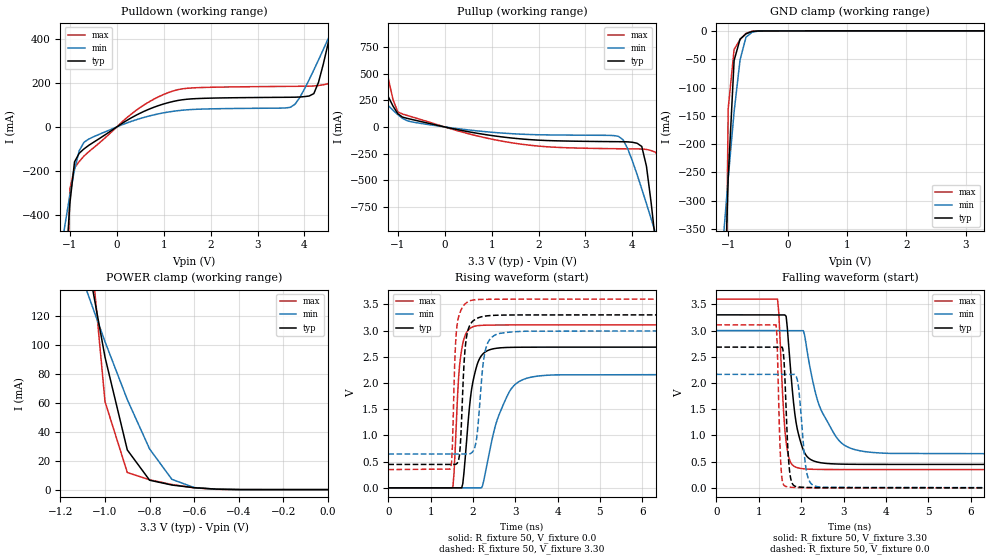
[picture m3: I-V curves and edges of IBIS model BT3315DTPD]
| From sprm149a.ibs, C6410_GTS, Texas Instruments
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[Model]   BT3315DTPD
Model_type   I/O
Vinh = 2.00
Vinl = 0.80
Enable   Active-Low
Polarity   Non-Inverting
| signals   A, GZ, Y
Vmeas = 1.5
|   typ   min   max
C_comp   1.6130p   1.5354p   1.7989p
|   typ   min   max
[Temperature Range]   25   -40   125
|   typ   min   max
[Voltage Range]   3.30V   3.00V   3.60V
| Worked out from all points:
|   slope of the pulldown table from 0 to 0.495 V, typ, clamps not added: 7.97 ohm
|   slope of the pullup table from 0 to 0.495 V, typ, clamps not added: 11.2 ohm
|   GND clamp passes 1 mA (typ) near -0.60 V on its own axis
|   POWER clamp passes 1 mA (typ) near -0.57 V on its own axis
|   rising waveform, R_fixture 50, V_fixture 0.0: 20-80 % time 219ps typ, 469ps min, 132ps max; typ from 0 V to 2.69 V
|   falling waveform, R_fixture 50, V_fixture 3.30: 20-80 % time 235ps typ, 561ps min, 133ps max; typ from 3.3 V to 0.447 V
|   rising waveform, R_fixture 50, V_fixture 3.30: 20-80 % time 109ps typ, 160ps min, 84.2ps max; typ from 0.447 V to 3.3 V
|   falling waveform, R_fixture 50, V_fixture 0.0: 20-80 % time 89.5ps typ, 141ps min, 67.2ps max; typ from 2.69 V to 0 V
[Pulldown]
|   Voltage   I(typ)   I(min)   I(max)
-3.3V     -10.57A    -3.704A    -44.33A
-1.1V     -692.7mA   -440.2mA   -1.224A
-1V       -348.9mA   -310.5mA   -283mA
-900mV    -158.9mA   -194.3mA   -185.9mA
-700mV    -100.1mA   -70.15mA   -132.7mA
1V        104.5mA    64.15mA    147.5mA
3.7V      134.9mA    89.3mA     184.4mA
4.2V      151.5mA    259mA      186.1mA
4.6V      471.5mA    445.7mA    222.9mA
4.7V      570.4mA    493.5mA    367.2mA
4.8V      670.8mA    541.6mA    570.5mA
6.6V      2.55A      1.424A     4.92A
[GND_clamp]
|   Voltage   I(typ)   I(min)   I(max)
-3.3V     -10.46A    -3.63A     -44.21A
-1.1V     -613.6mA   -391.4mA   -1.123A
-1V       -261.2mA   -261.2mA   -137.9mA
-900mV    -52.12mA   -142.7mA   -32.7mA
-800mV    -14.54mA   -51.2mA    -15.3mA
-700mV    -5.175mA   -11.01mA   -4.371mA
-600mV    -1.021mA   -2.48mA    -553.4uA
-400mV    -41.03uA   -73.53uA   -56.54uA
3.3V      100.9uA    56.36uA    177.6uA
[Pullup]
|   Voltage   I(typ)   I(min)   I(max)
-3.3V     2.44A      1.204A     5.523A
-2.7V     1.811A     911.7mA    4.044A
-1.9V     980.1mA    525.4mA    2.088A
-1.5V     573.1mA    336.2mA    1.129A
-1.1V     195.1mA    156.3mA    255.9mA
-800mV    80.53mA    58.19mA    108mA
3.7V      -138.7mA   -87.83mA   -205mA
4.2V      -183.3mA   -582.4mA   -207.6mA
4.5V      -1.109A    -1.007A    -239.2mA
4.6V      -1.528A    -1.151A    -325.8mA
4.7V      -1.958A    -1.297A    -1.261A
6.6V      -10.56A    -4.136A    -38.31A
[POWER_clamp]
|   Voltage   I(typ)   I(min)   I(max)
-3.3V     2.436A     1.198A     5.522A
-1.1V     176.4mA    145.2mA    226.7mA
-1V       91.57mA    102.3mA    60.82mA
-900mV    27.41mA    62.23mA    11.8mA
-800mV    6.5mA      28.11mA    6.81mA
-700mV    3.158mA    7.093mA    3.523mA
-600mV    1.326mA    1.416mA    1.233mA
-500mV    313.8uA    312uA      181.6uA
0V        1pA        1pA        1pA
[Ramp]
|   I(typ)   I(min)   I(max)
dV/dt_r   1.611/0.219n   1.299/0.468n   1.865/0.132n
dV/dt_f   1.712/0.234n   1.413/0.562n   1.951/0.132n
[Rising Waveform]
R_fixture = 50
V_fixture = 0.0
|  pu_on
|  TIME   V(typ)   V(min)   V(max)
0s        1nV        11nV       1nV
1.526ns   938.3uV    158.3uV    19.43mV
1.656ns   938.3uV    392.6uV    2.051V
1.708ns   938.3uV    545.6uV    2.501V
1.76ns    79.62mV    867.3uV    2.754V
1.993ns   2.001V     959.6uV    3.071V
2.305ns   2.6V       337.9mV    3.103V
2.72ns    2.675V     1.593V     3.107V
3.239ns   2.683V     2.082V     3.108V
10ns      2.685V     2.165V     3.108V
[Falling Waveform]
R_fixture = 50
V_fixture = 3.30
V_fixture_min = 3.00
V_fixture_max = 3.60
|  pd_on
|  TIME   V(typ)   V(min)   V(max)
0s        3.3V       3V         3.6V
1.444ns   3.298V     3V         3.6V
1.589ns   3.298V     2.999V     1.421V
1.647ns   3.272V     2.998V     871.4mV
1.878ns   1.259V     2.998V     394.2mV
2.052ns   721.4mV    2.998V     364.6mV
2.197ns   555.4mV    2.35V      356.3mV
2.487ns   476.3mV    1.459V     351.2mV
3.181ns   449.9mV    751.3mV    349mV
10ns      447mV      645mV      348.6mV
[Rising Waveform]
R_fixture = 50
V_fixture = 3.30
V_fixture_min = 3.00
V_fixture_max = 3.60
|  pd_off
|  TIME   V(typ)   V(min)   V(max)
0s        447mV      644.9mV    348.6mV
1.458ns   447mV      645.3mV    358.8mV
1.625ns   467.7mV    645.3mV    3.108V
1.699ns   780.6mV    645.3mV    3.356V
1.81ns    2.614V     645.3mV    3.505V
1.921ns   3.093V     648mV      3.566V
2.087ns   3.23V      945.8mV    3.591V
2.291ns   3.277V     2.615V     3.596V
2.568ns   3.293V     2.932V     3.598V
10ns      3.3V       3V         3.6V
[Falling Waveform]
R_fixture = 50
V_fixture = 0.0
|  pu_off
|  TIME   V(typ)   V(min)   V(max)
0s        2.685V     2.165V     3.108V
1.408ns   2.684V     2.165V     3.108V
1.528ns   2.684V     2.164V     351.4mV
1.635ns   1.74V      2.164V     27.72mV
1.702ns   554.9mV    2.164V     15.66mV
1.769ns   131.1mV    2.164V     10.61mV
1.929ns   17.56mV    1.976V     5.239mV
2.142ns   7.953mV    251.8mV    2.369mV
2.329ns   4.561mV    33.16mV    1.403mV
10ns      259.2nV    3.875uV    131.1nV
